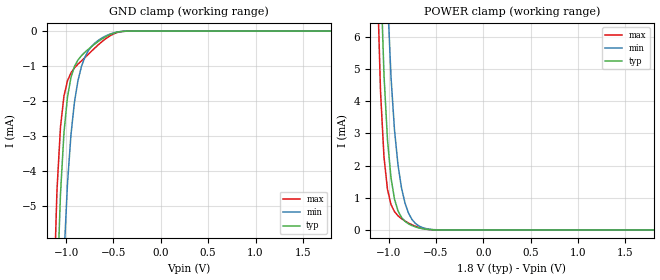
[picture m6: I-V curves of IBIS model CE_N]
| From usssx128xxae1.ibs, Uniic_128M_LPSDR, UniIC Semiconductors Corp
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|   Model CE_N
[Model] CE_N
Model_type Input
Vinl =  0.0V
Vinh =  1.800V
C_comp   0.580pF   0.575pF   0.585pF
[Model Spec]
Vinh   1.800V   1.400V   2.100V
Vinl   0.0V   -0.300V   0.400V
[Temperature Range]   25.000   0.125k   -40.000
[Voltage Range]   1.800V   1.620V   1.980V
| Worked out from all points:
|   GND clamp passes 1 mA (typ) near -0.91 V on its own axis
|   POWER clamp passes 1 mA (typ) near -0.94 V on its own axis
[GND_clamp]
|Voltage   I(typ)   I(min)   I(max)
-1.8V     -227.6mA   -264.4mA   -210.7mA
-1.134V   -11.9mA    -19.54mA   -7.897mA
-1.097V   -7.565mA   -13.86mA   -4.578mA
-1.06V    -4.683mA   -9.57mA    -2.756mA
-1.023V   -2.915mA   -6.495mA   -1.861mA
-986mV    -1.894mA   -4.381mA   -1.426mA
-949mV    -1.326mA   -2.966mA   -1.196mA
-875mV    -826.6uA   -1.417mA   -945.7uA
-764mV    -515.8uA   -555.9uA   -660.6uA
-616mV    -216.2uA   -188.2uA   -289.9uA
-357mV    -2.111uA   -3.116uA   -2.383uA
1.8V      0A         0A         0A
[POWER_clamp]
|Voltage   I(typ)   I(min)   I(max)
-1.8V     294.3mA    352.9mA    267.9mA
-1.123V   13.24mA    23.17mA    8.114mA
-1.086V   8.14mA     16.15mA    4.33mA
-1.049V   4.814mA    10.94mA    2.266mA
-1.012V   2.795mA    7.255mA    1.256mA
-975mV    1.621mA    4.757mA    791.4uA
-938mV    957.3uA    3.104mA    568.1uA
-901mV    591.9uA    2.018mA    440.7uA
-864mV    390.2uA    1.305mA    350.6uA
-790mV    192uA      522.8uA    215.4uA
-531mV    4.84uA     12.03uA    5.023uA
1.8V      0A         0A         0A
